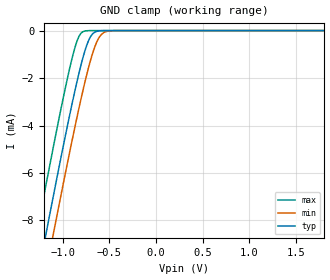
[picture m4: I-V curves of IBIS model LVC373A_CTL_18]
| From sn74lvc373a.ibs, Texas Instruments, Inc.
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[Model]   LVC373A_CTL_18
Model_type  Input
Vinl=0.5775
Vinh=1.2675
| variable   typ   min   max
C_comp   6.26pF   2.36pF   8.55pF
[Temperature Range]   40   100   -40
| Ambient temperature   25   85   -40
[Voltage range]   1.8   1.65   1.95
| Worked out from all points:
|   GND clamp passes 1 mA (typ) near -0.77 V on its own axis
[GND Clamp]
| LVC373A_CTL_18
|   Voltage   I(typ)   I(min)   I(max)
-5V       -90.43mA   -91.87mA   -88.61mA
-1.295V   -10.95mA   -12.54mA   -8.886mA
-1.26V    -10.22mA   -11.82mA   -8.161mA
-1.17V    -8.383mA   -9.982mA   -6.315mA
-1.095V   -6.868mA   -8.465mA   -4.803mA
-930mV    -3.652mA   -5.216mA   -1.678mA
-835mV    -1.957mA   -3.443mA   -332.7uA
-765mV    -899.4uA   -2.23mA    -22.13uA
-705mV    -284.6uA   -1.306mA   -1.254uA
-635mV    -34.23uA   -487.3uA   -41.86nA
-565mV    -2.862uA   -99.75uA   -1.396nA
1.8V      4.942pA    12.9pA     4.394pA
